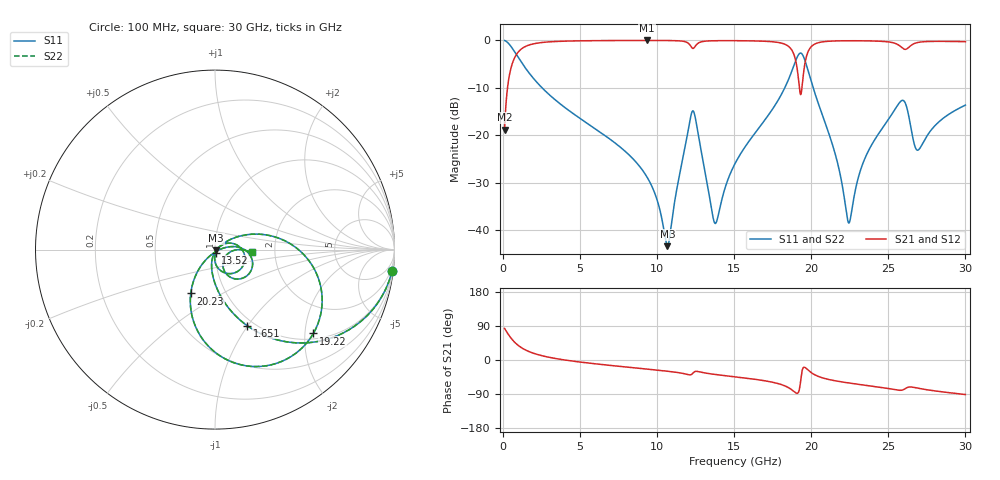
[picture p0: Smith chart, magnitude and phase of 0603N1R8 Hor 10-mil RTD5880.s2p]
# GHz S MA R 50
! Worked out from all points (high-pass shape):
!   3201 points, 100 MHz to 30 GHz, reference 50 ohm
!   highest |S21| = -0.05 dB at 9.341 GHz (marker M1); lowest = -18.8 dB at 100 MHz (marker M2)
!   |S21| within 3 dB of the highest: 858.8 MHz to 18.88 GHz (18.02 GHz wide, 183 % of centre); 19.72 GHz to end of sweep
!   lowest |S11| = -43.4 dB at 10.67 GHz (marker M3), VSWR 1.01, Z = 50.6 - j0.398 ohm
!   |S11| at or under -10 dB: 2.523 GHz to 18.28 GHz (15.76 GHz wide, 152 % of centre); 20.12 GHz to end of sweep
!   |S22| runs from -43.4 to -0.1 dB; largest |S21 - S12| = 0
!   S11 on the Smith chart (normalised r, x): 100 MHz: 1, -17; 1.651 GHz: 0.92, -0.99; 13.52 GHz: 1.01, -0.03; 19.22 GHz: 1.14, -2.21; 20.23 GHz: 0.68, -0.36; 30 GHz: 1.52, -0.05
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0.1  0.9934 -6.9  0.1145 83.1  0.1145 83.1  0.9934 -6.9
0.6045625  0.8197 -36.6  0.5722 53.4  0.5722 53.4  0.8197 -36.6
1.651063  0.4601 -67.1  0.8865 22.8  0.8865 22.8  0.4601 -67.1
5.089563  0.1463 -94.8  0.9865 -5.9  0.9865 -5.9  0.1463 -94.8
9.340969  0.03614 -107.0  0.9948 -24.0  0.9948 -24.0  0.03614 -107.0
10.06978  0.01892 -100.9  0.9945 -27.0  0.9945 -27.0  0.01892 -100.9
10.66778  0.006755 -35.7  0.9931 -29.6  0.9931 -29.6  0.006755 -35.7
12.29359  0.1795 -25.8  0.8226 -35.9  0.8226 -35.9  0.1795 -25.8
13.51763  0.01695 -73.0  0.9861 -36.8  0.9861 -36.8  0.01695 -73.0
13.84466  0.01215 -15.6  0.9886 -38.5  0.9886 -38.5  0.01215 -15.6
15.05  0.05008 35.2  0.9895 -44.3  0.9895 -44.3  0.05008 35.2
18.41375  0.3514 11.0  0.8866 -70.7  0.8866 -70.7  0.3514 11.0
19.21731  0.72 -40.4  0.331 -79.2  0.331 -79.2  0.72 -40.4
19.50697  0.665 -76.0  0.4654 -19.4  0.4654 -19.4  0.665 -76.0
20.03956  0.3487 -113.0  0.8695 -34.5  0.8695 -34.5  0.3487 -113.0
20.22644  0.2789 -119.0  0.9124 -39.1  0.9124 -39.1  0.2789 -119.0
22.43156  0.01184 -61.2  0.9879 -60.6  0.9879 -60.6  0.01184 -61.2
23.40331  0.05306 10.8  0.9863 -66.0  0.9863 -66.0  0.05306 10.8
25.01978  0.1477 3.2  0.9598 -75.4  0.9598 -75.4  0.1477 3.2
26.01022  0.2295 -40.0  0.808 -77.6  0.808 -77.6  0.2295 -40.0
26.92591  0.06949 -31.0  0.9481 -74.5  0.9481 -74.5  0.06949 -31.0
30  0.2072 -4.4  0.966 -91.1  0.966 -91.1  0.2072 -4.4
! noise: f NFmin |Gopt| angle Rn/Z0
0.1  0.0004534  0.9494  0.9883  0.002012
3.417  0.004037  0.8101  9.903  0.004398
6.743  0.006872  0.784  19.04  0.006357
10.06  0.01068  0.793  28.04  0.01003
13.39  0.02104  0.8567  37.04  0.02824
16.7  0.02097  0.8256  45.71  0.02149
20.03  0.05835  0.9219  54.57  0.1306
23.35  0.02414  0.7969  62.84  0.01799
26.67  0.06733  0.9126  71.14  0.1123
30  0.02739  0.7783  78.78  0.01526
